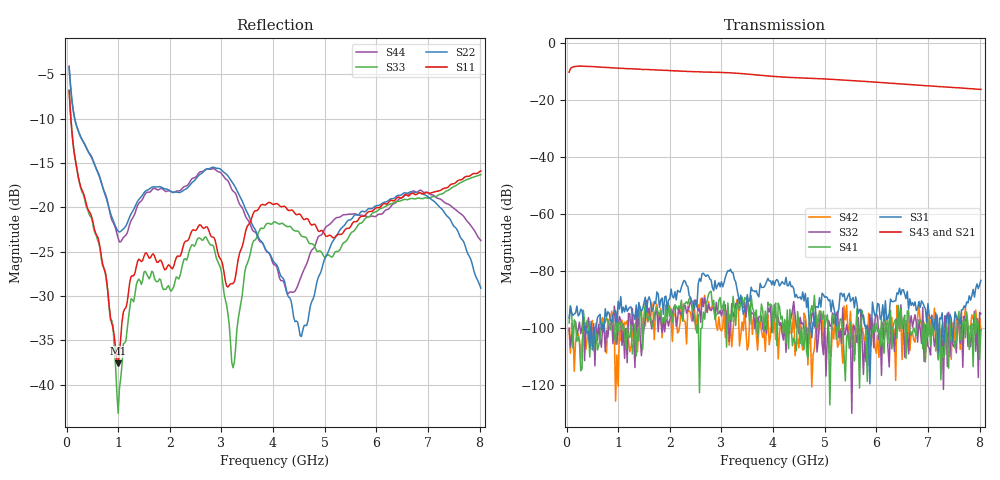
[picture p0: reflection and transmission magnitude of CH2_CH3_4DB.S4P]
!Agilent Technologies,E5071C,MY46316741,A.11.02
!Date: Thu May 28 14:39:54 2026
!Data & Calibration Information:
!1:CH2 INPUT 2:CH2 OUTPUT 3:CH3 INPUT 4:CH3 OUTPUT
!Freq	S11:SOLT4(ON)	S12:SOLT4(ON)	S13:SOLT4(ON)	S14:SOLT4(ON)
!	S21:SOLT4(ON)	S22:SOLT4(ON)	S23:SOLT4(ON)	S24:SOLT4(ON)
!	S31:SOLT4(ON)	S32:SOLT4(ON)	S33:SOLT4(ON)	S34:SOLT4(ON)
!	S41:SOLT4(ON)	S42:SOLT4(ON)	S43:SOLT4(ON)	S44:SOLT4(ON)
!PortZ  Port1:50+j0  Port2:50+j0  Port3:50+j0  Port4:50+j0
!Above PortZ is port z conversion or system Z0 setting when saving the data.
!When reading, reference impedance value at option line is always used.
# Hz S dB R 50
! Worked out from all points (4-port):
!   320 points, 50 MHz to 8.025 GHz, reference 50 ohm
!   strongest paths, dB at 50 MHz, 2.05 GHz, 4.05 GHz, 6.05 GHz, 8.025 GHz:
!     S43: -10.2, -9.7, -11.8, -13.8, -16.3
!     S21: -10.3, -9.8, -12.0, -14.0, -16.5
!     S31: -96.7, -89.1, -83.6, -91.8, -83.4
!     S41: -98.4, -98.2, -91.4, -100.7, -100.8
!     S32: -100.2, -94.9, -96.5, -104.2, -95.2
!     S42: -100.7, -104.9, -104.2, -110.4, -100.9
!   lowest |S11| = -37.6 dB at 1 GHz (marker M1), VSWR 1.03, Z = 49.2 - j1.01 ohm
!   |S11| at or under -10 dB: 84.38 MHz to end of sweep
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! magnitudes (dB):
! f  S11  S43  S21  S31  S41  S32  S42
! 50 MHz  -6.8  -10.2  -10.3  -96.7  -98.4  -100.2  -100.7
! 1 GHz  -37.6  -8.8  -9.0  -90.8  -101.4  -99.0  -120.6
! 1.525 GHz  -25.2  -9.3  -9.4  -89.3  -91.4  -97.3  -99.5
! 3.225 GHz  -28.6  -10.5  -10.7  -80.7  -89.0  -96.1  -101.0
! 4.55 GHz  -21.0  -12.3  -12.5  -90.1  -99.7  -98.7  -105.2
! 6.55 GHz  -18.6  -14.5  -14.7  -88.3  -95.6  -110.4  -99.7
! 8.025 GHz  -15.9  -16.3  -16.5  -83.4  -100.8  -95.2  -100.9
